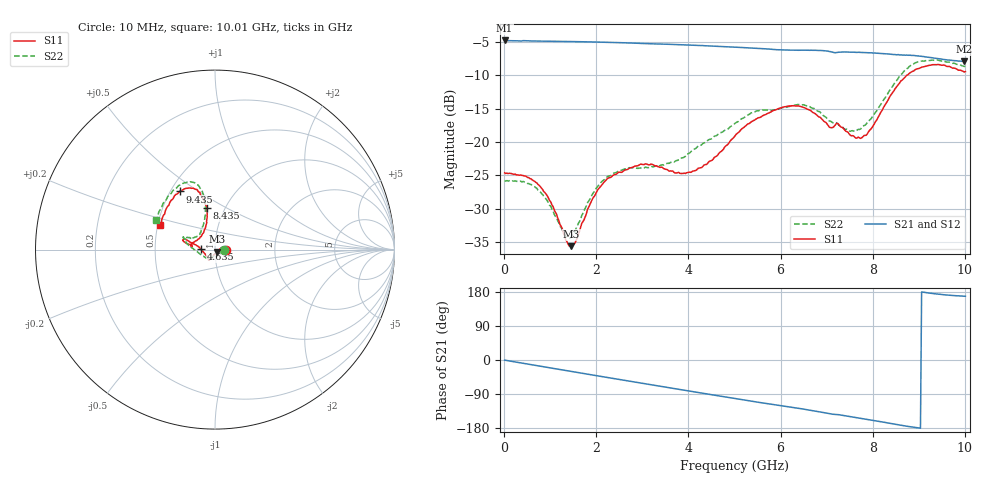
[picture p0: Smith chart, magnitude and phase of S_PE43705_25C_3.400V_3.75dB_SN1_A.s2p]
! Device ID: PE43705
! Serial: 1
! Insertion: A
! Impedance: 50 ohm
! Temp: 25C
! VDD: 3.400V
! Attenuation Step: 3.75dB
#  Hz  S  RI  R  50
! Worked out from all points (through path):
!   401 points, 10 MHz to 10.01 GHz, reference 50 ohm
!   highest |S21| = -4.81 dB at 10 MHz (marker M1); lowest = -7.9 dB at 9.985 GHz (marker M2)
!   group delay of S21, straight-line fit = 54.5 ps
!   lowest |S11| = -35.6 dB at 1.46 GHz (marker M3), VSWR 1.03, Z = 51.1 - j1.24 ohm
!   |S11| at or under -10 dB: start of sweep to 8.745 GHz
!   |S22| runs from -34.4 to -7.7 dB; largest |S21 - S12| = 0.0048
!   S11 on the Smith chart (normalised r, x): 10 MHz: 1.12, -0.00; 4.635 GHz: 0.85, +0.01; 8.435 GHz: 0.82, +0.40; 9.435 GHz: 0.56, +0.42; 10.01 GHz: 0.51, +0.16
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1e7  0.0587 -0.000258  0.5746 -0.00288  0.575 -0.00267  0.0514 -9.02e-05
7.6e8  0.045 0.0147  0.547 -0.155  0.547 -0.1547  0.0409 0.0124
1.31e9  0.0196 -0.00372  0.5031 -0.2573  0.5032 -0.257  0.0189 -0.00766
1.46e9  0.0114 -0.0121  0.4874 -0.2834  0.4876 -0.2835  0.0116 -0.0158
1.685e9  0.000285 -0.0247  0.4615 -0.3207  0.4615 -0.3207  0.000707 -0.0282
2.235e9  -0.0205 -0.0489  0.386 -0.4007  0.3863 -0.4004  -0.0229 -0.0499
2.935e9  -0.0337 -0.0584  0.2712 -0.4751  0.2719 -0.4752  -0.0399 -0.0498
3.36e9  -0.0359 -0.0542  0.1959 -0.5037  0.1966 -0.5032  -0.0461 -0.0473
3.985e9  -0.0511 -0.0296  0.0801 -0.5255  0.0806 -0.5248  -0.0755 -0.0303
4.635e9  -0.0796 0.00471  -0.0389 -0.5177  -0.038 -0.5176  -0.1135 -0.00159
5.01e9  -0.1079 0.0269  -0.103 -0.5011  -0.1024 -0.5014  -0.1368 0.0161
6.01e9  -0.1707 0.0575  -0.2479 -0.4211  -0.2461 -0.4219  -0.1693 0.0596
6.685e9  -0.1636 0.0374  -0.3339 -0.3519  -0.334 -0.3515  -0.1649 0.0706
7.435e9  -0.1099 0.0471  -0.3989 -0.2503  -0.3982 -0.2512  -0.0994 0.075
7.71e9  -0.0804 0.0711  -0.419 -0.2087  -0.4181 -0.2098  -0.0808 0.094
7.935e9  -0.0598 0.1071  -0.4311 -0.1737  -0.4307 -0.1762  -0.0694 0.1287
8.36e9  -0.044 0.2108  -0.4424 -0.104  -0.4413 -0.1064  -0.0539 0.2353
8.435e9  -0.0469 0.2308  -0.4424 -0.0912  -0.4422 -0.0929  -0.0545 0.2573
8.885e9  -0.0946 0.3256  -0.4437 -0.02  -0.4406 -0.022  -0.1083 0.3677
9.435e9  -0.1977 0.324  -0.4164 0.0463  -0.4154 0.0467  -0.2091 0.3497
9.985e9  -0.2991 0.1482  -0.3926 0.081  -0.3939 0.0807  -0.3223 0.1758
1.001e10  -0.3062 0.1381  -0.3935 0.0825  -0.3957 0.0816  -0.3297 0.1638
